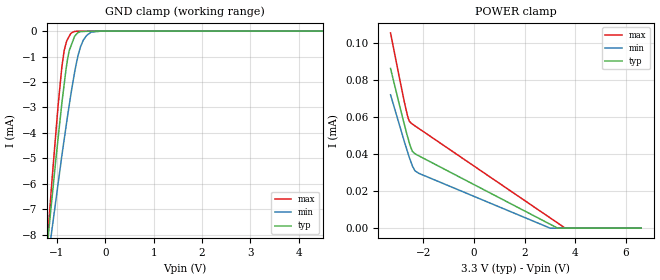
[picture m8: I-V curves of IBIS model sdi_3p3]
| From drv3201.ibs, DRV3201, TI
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|   sdi_3p3 Model
[Model]   sdi_3p3
Model_type   Input
Vinl = 0.99
Vinh = 2.31
|   typ   min   max
|   (nom PVT)   (fast PVT)   (slow PVT)
 C_comp   4.837e-13   4.556e-13   5.145e-13
| Where nom  PVT is Nominal Process, 3.3V, 27C
|   Fast PVT is Strong Process,  3.6V, -40C
|   Slow PVT is Weak Process,   3V, 150C
[Voltage Range]   3.3   3   3.6
|Junction Temperature
[Temperature Range]   27   150   -40
[Power Clamp Reference]   3.3   3   3.6
[GND Clamp Reference]   0   0   0
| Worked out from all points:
|   GND clamp passes 1 mA (typ) near -0.77 V on its own axis
[GND Clamp]
|   Voltage   I(typ)   I(min)   I(max)
-3.3V     -51.89mA   -41.44mA   -64.03mA
-1.181V   -8.107mA   -8.932mA   -7.874mA
-1.094V   -6.445mA   -7.697mA   -5.706mA
-975.6mV  -4.23mA    -6.011mA   -2.948mA
-896.4mV  -2.821mA   -4.887mA   -1.399mA
-849.6mV  -2.098mA   -4.266mA   -769uA
-745.8mV  -770.9uA   -2.923mA   -205.4uA
-633.6mV  -206.9uA   -1.624mA   -11.36uA
-561mV    -61.22uA   -952.7uA   -7.09uA
-456mV    -15uA      -365.3uA   -4.259uA
-285mV    -2.039uA   -39.79uA   -2.659uA
6.6V      0A         0A         0A
[POWER Clamp]
|   Voltage   I(typ)   I(min)   I(max)
-3.3V     86.47uA    72.2uA     105.7uA
-2.966V   67.71uA    56.69uA    82.52uA
-2.758V   56.33uA    46.98uA    68.53uA
-2.635V   49.93uA    41.61uA    61.14uA
-2.56V    46.24uA    38.31uA    57.96uA
-2.462V   42.44uA    34.65uA    56.57uA
-2.337V   40.35uA    31.12uA    55.4uA
-2.19V    39.21uA    29.73uA    54.03uA
2.997V    2.164uA    19.13nA    5.626uA
3.3V      0A         0A         2.799uA
3.596V    0A         0A         33.59nA
6.6V      0A         0A         0A
